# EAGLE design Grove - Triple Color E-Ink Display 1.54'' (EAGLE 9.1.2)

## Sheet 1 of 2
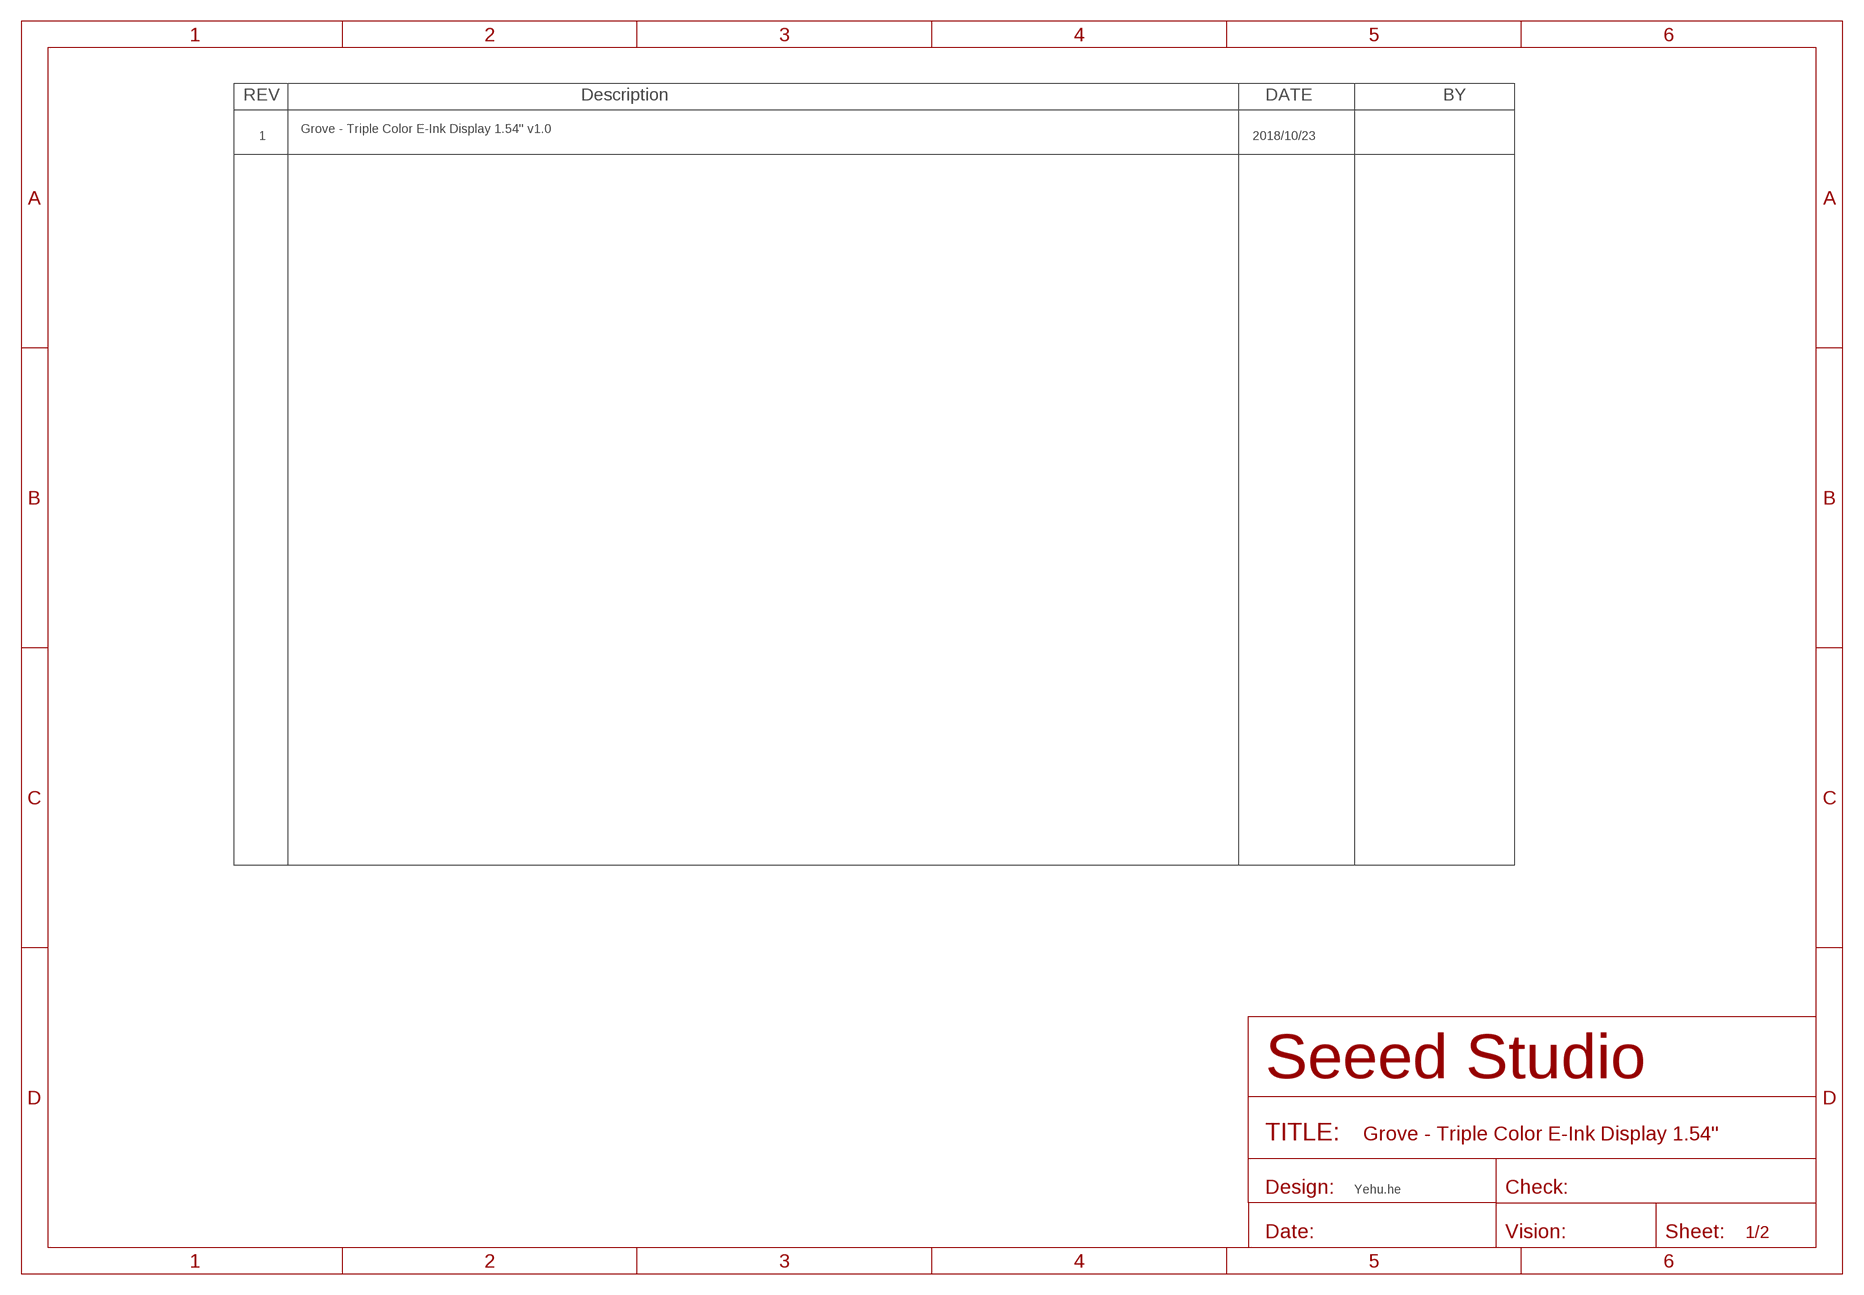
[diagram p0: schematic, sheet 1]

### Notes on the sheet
- Grove - Triple Color E-Ink Display 1.54'' v1.0
- 1 | 2018/10/23
- Yehu.he

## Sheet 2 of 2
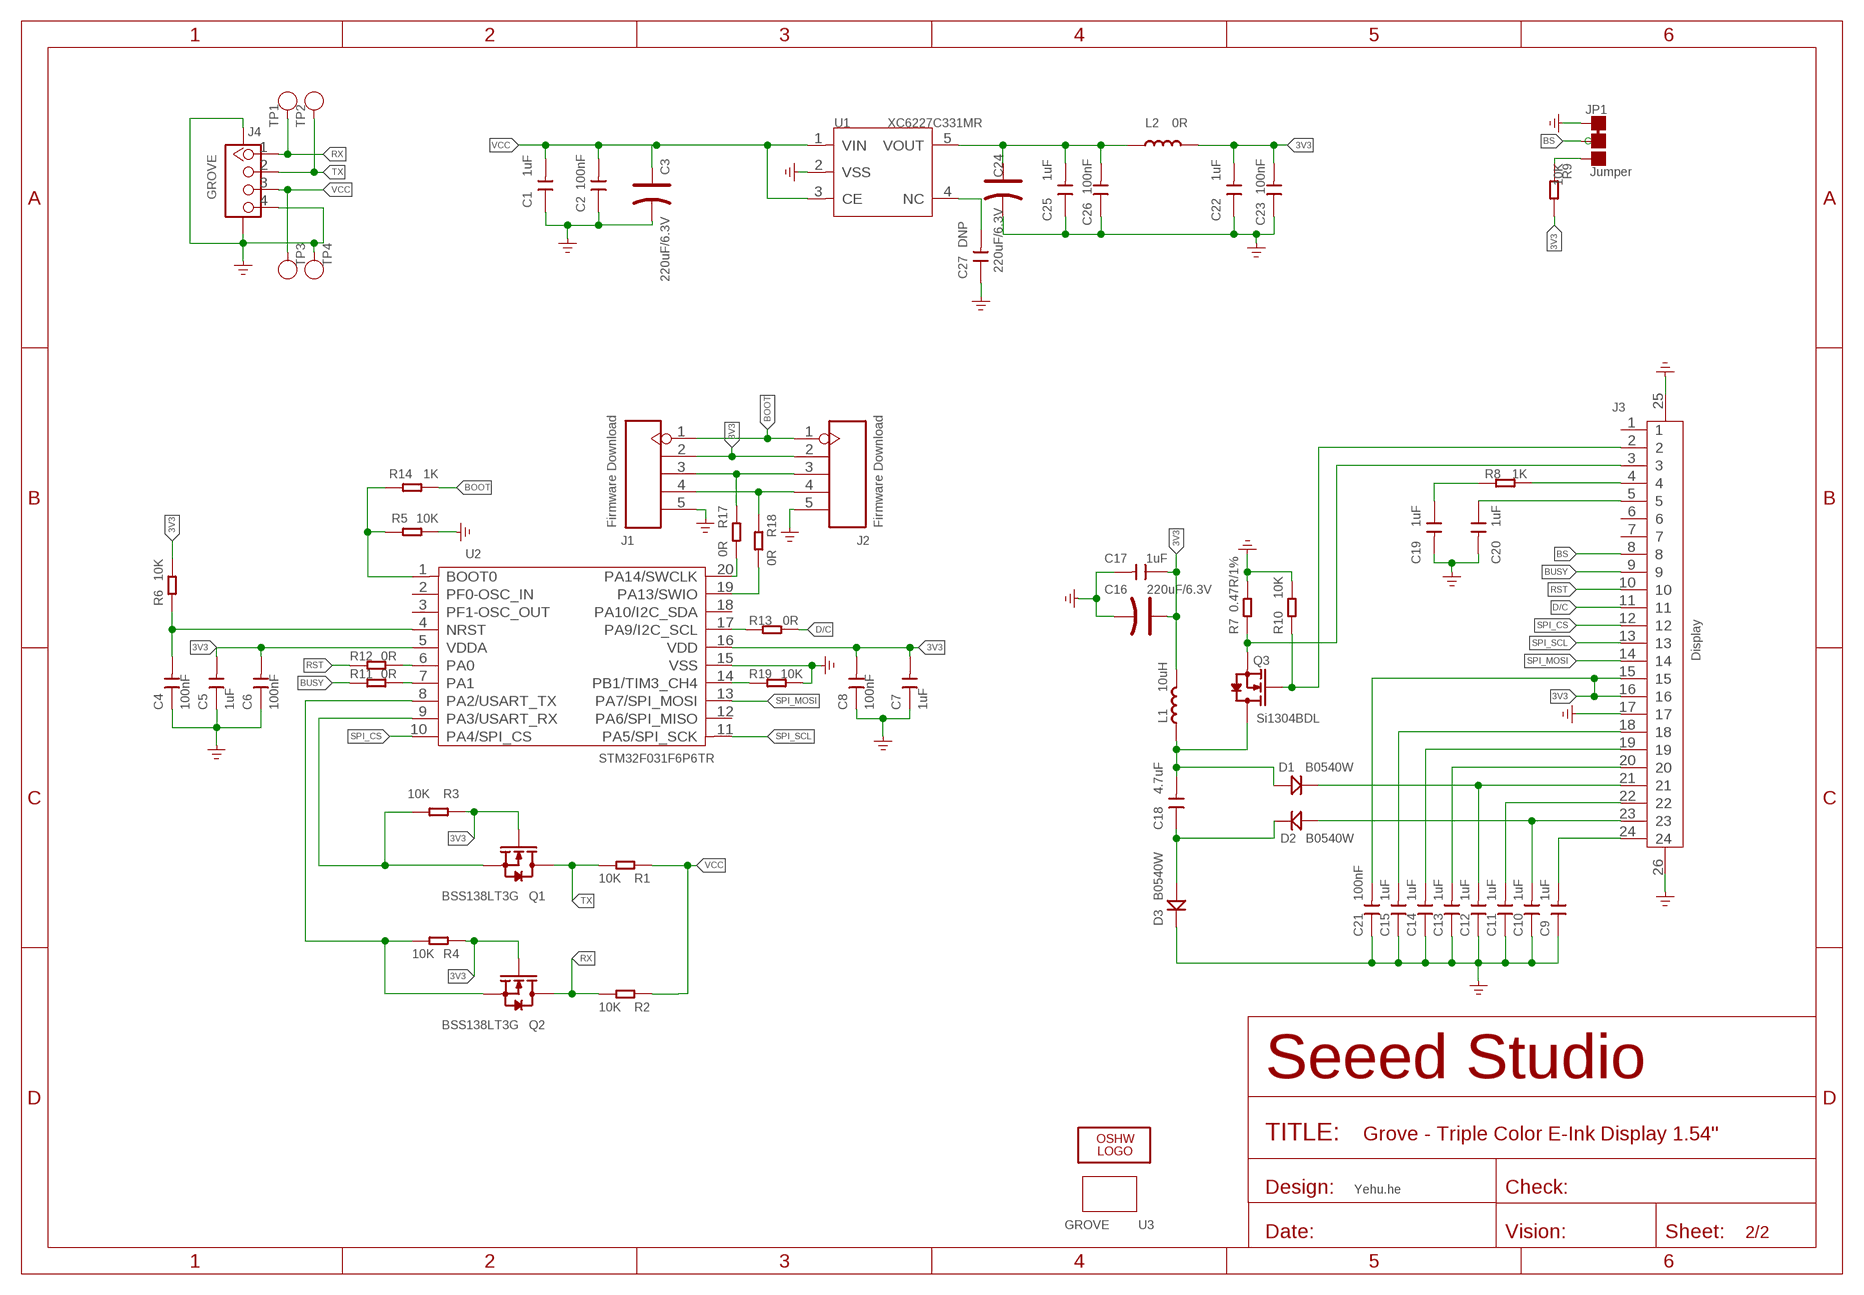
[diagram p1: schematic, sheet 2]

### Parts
C1  1uF  CAP-0603  [C0603]
C2  100nF  CAP-0603  [C0603]
C3  220uF/6.3V  CAP-POLAR-AVX-B  [AVX-B]
C4  100nF  CAP-0603  [C0603]
C5  1uF  CAP-0603  [C0603]
C6  100nF  CAP-0603  [C0603]
C7  1uF  CAP-0603  [C0603]
C8  100nF  CAP-0603  [C0603]
C9  1uF  CAP-0603  [C0603]
C10  1uF  CAP-0603  [C0603]
C11  1uF  CAP-0603  [C0603]
C12  1uF  CAP-0603  [C0603]
C13  1uF  CAP-0603  [C0603]
C14  1uF  CAP-0603  [C0603]
C15  1uF  CAP-0603  [C0603]
C16  220uF/6.3V  CAP-POLAR-AVX-B  [AVX-B]
C17  1uF  CAP-0603  [C0603]
C18  4.7uF  CAP-0805  [C0805]
C19  1uF  CAP-0603  [C0603]
C20  1uF  CAP-0603  [C0603]
C21  100nF  CAP-0603  [C0603]
C22  1uF  CAP-0805  [C0805]
C23  100nF  CAP-0603  [C0603]
C24  220uF/6.3V  CAP-POLAR-AVX-B  [AVX-B]
C25  1uF  CAP-0805  [C0805]
C26  100nF  CAP-0603  [C0603]
C27  DNP  CAP-0603  [C0603]
D1  B0540W  DIODE'0805'  [SOD-323]
D2  B0540W  DIODE'0805'  [SOD-323]
D3  B0540W  DIODE'0805'  [SOD-323]
J1  Firmware Download  HEADER-5P-SMD2.54  [H5-SMD-2.54]
J2  Firmware Download  HEADER-5P-SMD2.54  [H5-SMD-2.54]
J3  Display  FPC-CONNECTOR-24P  [FPCB24-SMD-0.5-17.6X5.0X2MM]
J4  GROVE  GROVE-CONNECTOR-SMD'90D'  [HW4-SMD-2.0-90D]
JP1  Jumper  JP-3P-SHORT  [3P-SMD-SHORT]
L1  10uH  INDUCTOR/FERRITE-BEAD5040S  [L5040S]
L2  0R  INDUCTOR/FERRITE-BEAD'0805'  [L0805]
LOGO2  LOGO-OSHW-FILLX0200-NT  [OSHW_FILLX200_NOTEXT]
Q1  BSS138LT3G  MOSFET-N'SI1304BDL'  [SOT-323]
Q2  BSS138LT3G  MOSFET-N'SI1304BDL'  [SOT-323]
Q3  Si1304BDL  MOSFET-N'SI1304BDL'  [SOT-323]
R1  10K  RES-0603  [R0603]
R2  10K  RES-0603  [R0603]
R3  10K  RES-0603  [R0603]
R4  10K  RES-0603  [R0603]
R5  10K  RES-0603  [R0603]
R6  10K  RES-0603  [R0603]
R7  0.47R/1%  RES-0603  [R0603]
R8  1K  RES-0603  [R0603]
R9  10K  RES-0603  [R0603]
R10  10K  RES-0603  [R0603]
R11  0R  RES-0603  [R0603]
R12  0R  RES-0603  [R0603]
R13  0R  RES-0603  [R0603]
R14  1K  RES-0603  [R0603]
R17  0R  RES-0603  [R0603]
R18  0R  RES-0603  [R0603]
R19  10K  RES-0603  [R0603]
TP1  Test  TEST-POINT'4545'  [TP-D45MIL]
TP2  Test  TEST-POINT'4545'  [TP-D45MIL]
TP3  Test  TEST-POINT'4545'  [TP-D45MIL]
TP4  Test  TEST-POINT'4545'  [TP-D45MIL]
U1  XC6227C331MR  PMIC-LDO-XC6210  [SOT-23-5]
U2  STM32F031F6P6TR  MCU-STM32F030  [TSSOP20-0.65-6.5X4.4MM]
U3  GROVE  GROVE'2X2U'  [GROVE-2*2-DRILL-DIM]

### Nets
3V3: C5.2 C6.2 C7.2 C8.2 C16.+ C17.1 C21.2 C22.2 C23.2 J1.2 J2.2 J3.15 J3.16 L1.2 L2.2 Q1.1(G) Q2.1(G) R3.2 R4.2 R6.1 R9.2 U2.5(VDDA) U2.16(VDD)
123: C24.+ C25.2 C26.2 L2.1 U1.5(VOUT)
BOOT: J1.1 J2.1 R14.1
BS: J3.8 JP1.MM(C)
BUSY: J3.9 R11.1
D/C: J3.11 R13.1
GDR: J3.2 Q3.1(G) R10.1
GND: C1.1 C2.1 C3.- C4.1 C5.1 C6.1 C7.1 C8.1 C9.1 C10.1 C11.1 C12.1 C13.1 C14.1 C15.1 C16.- C17.2 C19.2 C20.2 C21.1 C22.1 C23.1 C24.- C25.1 C26.1 C27.1 D3.- J1.5 J2.5 J3.17 J3.25(P1) J3.26(P2) J4.4 J4.SS1 J4.SS2 JP1.11(L) R5.1 R7.2 R10.2 R19.1 TP4.T U1.2(VSS) U2.15(VSS) ; supply symbol labelled GND_POWER
N$1: R11.2 U2.7(PA1)
N$2: R12.2 U2.6(PA0)
N$3: R13.2 U2.17(PA9/I2C_SCL)
N$4: J1.3 J2.3 R17.1
N$5: R5.2 R14.2 U2.1(BOOT0)
N$6: R19.2 U2.14(PB1/TIM3_CH4)
N$7: C27.2 U1.4(NC)
N$8: C4.2 R6.2 U2.4(NRST)
N$9: C18.1 D2.- D3.+
N$10: J1.4 J2.4 R18.1
N$11: C18.2 D1.+ L1.1 Q3.3(D)
N$12: C19.1 R8.2
N$13: R17.2 U2.20(PA14/SWCLK)
N$14: R18.2 U2.19(PA13/SWIO)
N$22: C15.2 J3.18
N$23: C14.2 J3.19
N$24: C13.2 J3.20
N$25: C12.2 D1.- J3.21
N$26: C11.2 J3.22
N$27: C10.2 D2.+ J3.23
N$28: JP1.00(R) R9.1
RESE: J3.3 Q3.2(S) R7.1
RST: J3.10 R12.1
RX: J4.1 Q2.3(D) R2.1 TP1.T
SCL_3V3: Q1.2(S) R3.1 U2.9(PA3/USART_RX)
SDA_3V3: Q2.2(S) R4.1 U2.8(PA2/USART_TX)
SPI_CS: J3.12 U2.10(PA4/SPI_CS)
SPI_MOSI: J3.14 U2.13(PA7/SPI_MOSI)
SPI_SCL: J3.13 U2.11(PA5/SPI_SCK)
TX: J4.2 Q1.3(D) R1.1 TP2.T
VCC: C1.2 C2.2 C3.+ J4.3 R1.2 R2.2 TP3.T U1.1(VIN) U1.3(CE)
VCOM: C9.2 J3.24
VGH: C20.1 J3.5
VGL: J3.4 R8.1
Unconnected: J3.1 J3.6 J3.7 U2.2(PF0-OSC_IN) U2.3(PF1-OSC_OUT) U2.12(PA6/SPI_MISO) U2.18(PA10/I2C_SDA)

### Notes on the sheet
- Yehu.he

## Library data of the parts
C1 C2 C4-C15 C17-C23 C25-C27 = Discrete-new:CAP: Ceramic Capacitors
C3 C16 C24 = Discrete-new:CAP-POLAR: Electrolytic Capacitors,Tantalum Capacitors and Super Capacitors
D1-D3 = Discrete-new:DIODE*
J1 J2 = Connector-new:HEADER-5P
J3 = Connector-new:FPC-CONNECTOR-24P
J4 = Connector-new:GROVE-CONNECTOR-SMD: 4P-SMD-2.0:320110030;4P-SMD-2.0-90D:320110032
JP1 = Discrete-new:JP-3P-SHORT
L1 L2 = Discrete-new:INDUCTOR/FERRITE-BEAD
LOGO2 = logo:LOGO-OSHW-FILL; PARTNO: DNP
Q1-Q3 = Discrete-new:MOSFET-N: IRLL014: http://www.vishay.com/docs/91319/sihll014.pdf
R1-R14 R17-R19 = Discrete-new:RES
TP1-TP4 = Discrete-new:TEST-POINT; PARTNO: DNP
U1 = IC-new:PMIC-LDO-XC6210
U2 = IC-new:MCU-STM32F030
U3 = moudle-new:GROVE

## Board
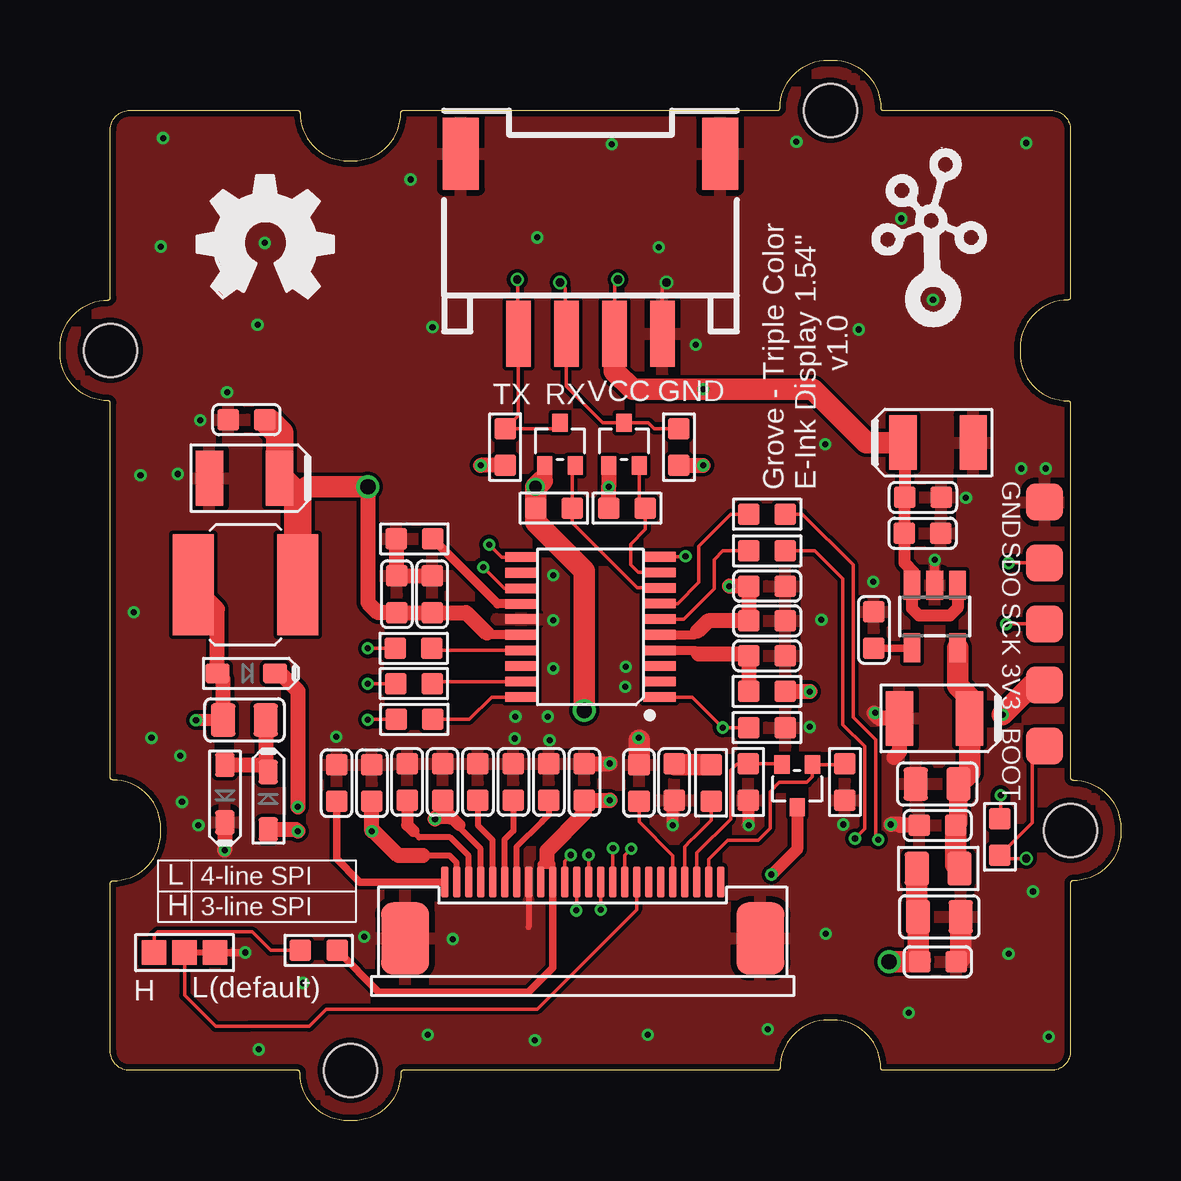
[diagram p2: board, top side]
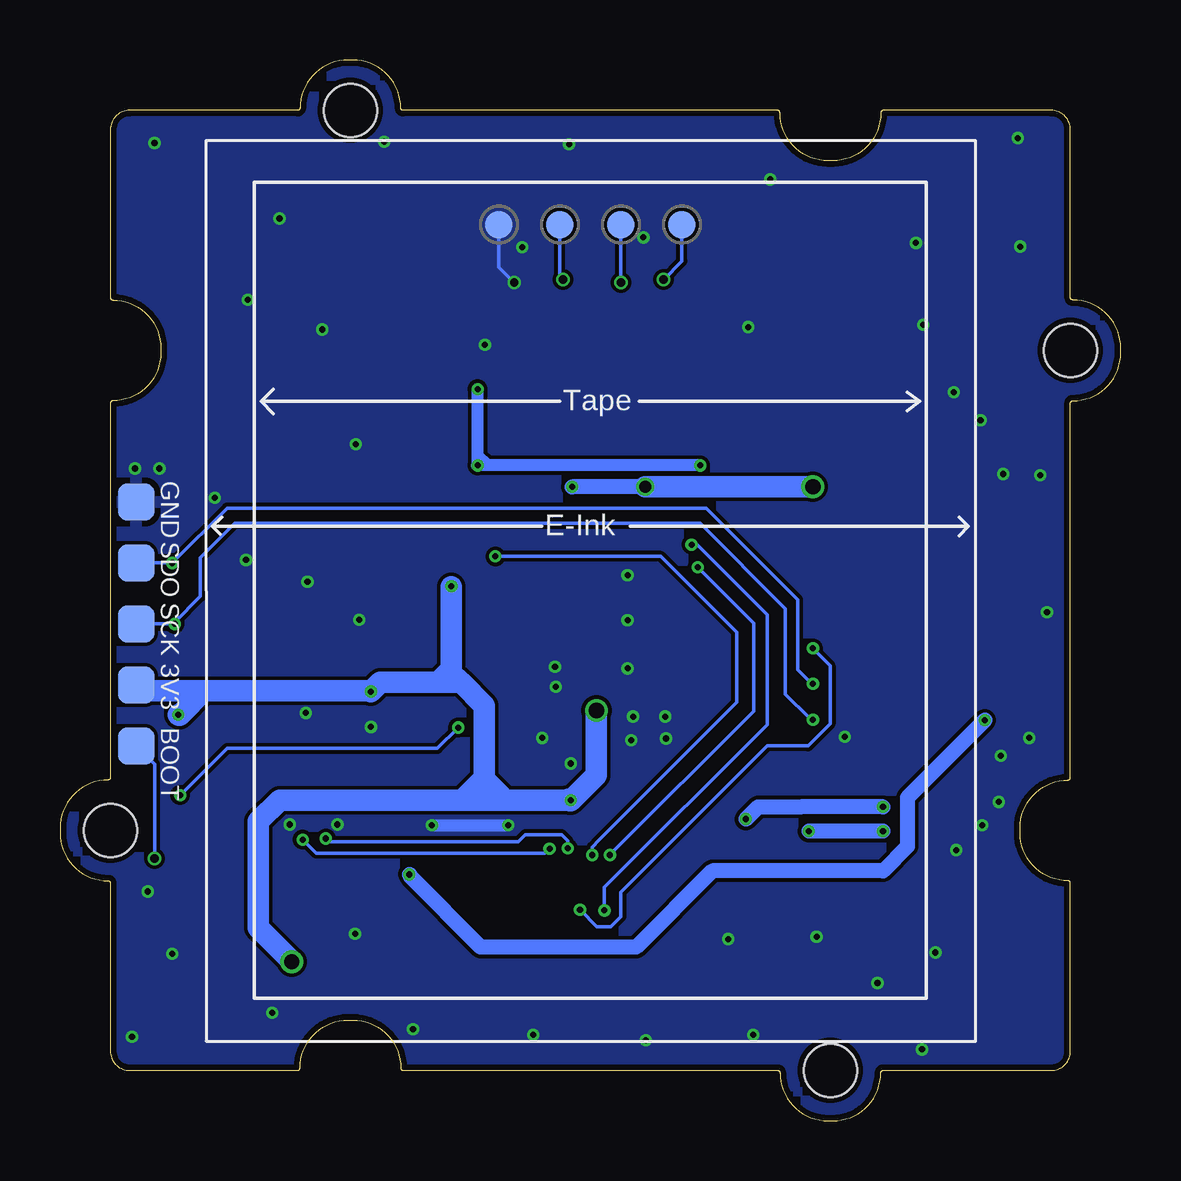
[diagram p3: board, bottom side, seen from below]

Size 44.2 x 44.2 mm. Coordinates in mm from the lower left corner, seen from the top.
Copper layers (1*16): Top 0.035mm / dielectric 1.5mm / Bottom 0.035mm
Design rules "SeeedStudio_2layer_DRU_no_angle_20140221": minimum track width 1mil, minimum drill 10mil, track to track 6mil, track to pad 6mil, pad to pad 6mil, via to via 6mil, smd to smd 0mil, copper to edge 10mil, drill to drill 10mil, minimum pad ring 4mil, minimum via ring 4mil, stop-mask expansion 2mil, vias tented up to drill 25mil, thermal gap 10mil

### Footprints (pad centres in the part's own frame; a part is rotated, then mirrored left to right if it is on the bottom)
C0603 = smd 0.889 x 0.889: 1 -0.762,0; 2 0.762,0
AVX-B = smd 1.143 x 2.286: + 1.46,0; - -1.46,0
C0805 = smd 1.016 x 1.397: 1 -0.889,0; 2 0.889,0
SOD-323 = smd 1 x 0.8: + 1.2,0; - -1.2,0
H5-SMD-2.54 = smd 1.524 x 1.524: 1 0,5.08; 2 0,2.54; 3 0,0; 4 0,-2.54; 5 0,-5.08
FPCB24-SMD-0.5-17.6X5.0X2MM = smd 0.3 x 1.3: 1 5.75,0; 2 5.25,0; 3 4.75,0; 4 4.25,0; 5 3.75,0; 6 3.25,0; 7 2.75,0; 8 2.25,0; 9 1.75,0; 10 1.25,0; 11 0.75,0; 12 0.25,0; 13 -0.25,0; 14 -0.75,0; 15 -1.25,0; 16 -1.75,0; 17 -2.25,0; 18 -2.75,0; 19 -3.25,0; 20 -3.75,0; 21 -4.25,0; 22 -4.75,0; 23 -5.25,0; 24 -5.75,0 | smd 2 x 3: 25 -7.4,-2.35; 26 7.4,-2.35
HW4-SMD-2.0-90D = smd 1.01 x 2.74: 1 -3,-0.1; 2 -1,-0.1; 3 1,-0.1; 4 3,-0.1 | smd 1.5 x 3: SS1 -5.4,7.4; SS2 5.4,7.4
3P-SMD-SHORT = smd 1.016 x 1.016: 00 -1.27,0; 11 1.27,0; MM 0,0
L5040S = smd 1.7 x 4.2: 1 -2.175,0; 2 2.175,0
L0805 = smd 1.016 x 1.397: 1 -0.889,0; 2 0.889,0
SOT-323 = smd 0.762 x 0.635: 1 0.889,-0.635; 2 0.889,0.635; 3 -0.889,0
R0603 = smd 0.889 x 0.889: 1 -0.762,0; 2 0.762,0
TP-D45MIL = smd 1.143 x 1.143: T 0,0
SOT-23-5 = smd 0.69 x 1.2: 1 -0.95,-1.3; 2 0,-1.3; 3 0.95,-1.3; 4 0.95,1.3; 5 -0.95,1.3
TSSOP20-0.65-6.5X4.4MM = smd 0.4 x 1.35: 1 -2.925,-2.875; 2 -2.275,-2.875; 3 -1.625,-2.875; 4 -0.975,-2.875; 5 -0.325,-2.875; 6 0.325,-2.875; 7 0.975,-2.875; 8 1.625,-2.875; 9 2.275,-2.875; 10 2.925,-2.875; 11 2.91,2.875; 12 2.26,2.875; 13 1.61,2.875; 14 0.96,2.875; 15 0.325,2.875; 16 -0.325,2.875; 17 -0.975,2.875; 18 -1.625,2.875; 19 -2.275,2.875; 20 -2.925,2.875
GROVE-2*2-DRILL-DIM = hole 2.2: 10,20; -20,10; -10,-20; 20,-10

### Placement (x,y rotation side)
C1  35.94,24.48 180 top
C2  35.96,25.97 180 top
C3  36.59,28.26 180 top
C4  29.46,19.37 180 top
C5  29.47,20.83 180 top
C6  29.47,22.28 180 top
C7  14.03,21.94 270 top
C8  15.51,21.94 270 top
C9  11.52,14.07 270 top
C10  13,14.07 270 top
C11  14.47,14.12 270 top
C12  15.94,14.12 270 top
C13  17.42,14.12 270 top
C14  18.89,14.12 270 top
C15  20.37,14.12 270 top
C16  7.69,26.78 0 top
C17  7.77,29.22 180 top
C18  7.69,16.7 180 top
C19  25.59,14.12 270 top
C20  24.12,14.08 90 top
C21  21.85,14.12 270 top
C22  36.64,8.5 180 top
C23  36.58,6.62 180 top
C24  36.44,16.77 0 top
C25  36.55,14.03 0 top
C26  36.56,12.31 0 top
C27  33.91,20.45 270 top
D1  7.76,18.64 180 top
D2  8.68,13.34 270 top
D3  6.87,13.63 90 top
J1  41.02,20.7 180 bottom
J2  41.02,20.7 180 top
J3  21.78,9.95 0 top
J4  22.1,32.9 0 top
JP1  5.19,7 0 top
L1  7.73,22.33 0 top
L2  36.59,10.51 180 top
LOGO2  5.72,34.29 0 top
Q1  23.5,28.2 270 top
Q2  20.83,28.2 270 top
Q3  30.71,13.96 90 top
R1  25.78,28.07 270 top
R2  18.54,28.07 270 top
R3  23.62,25.53 180 top
R4  20.58,25.53 180 top
R5  29.46,16.39 180 top
R6  29.46,17.89 180 top
R7  28.68,14.12 270 top
R8  27.13,14.08 90 top
R9  10.78,7.1 0 top
R10  32.7,14.12 270 top
R11  29.47,25.28 180 top
R12  29.47,23.75 180 top
R13  14.73,19.69 0 top
R14  39.16,11.83 90 top
R17  14.76,16.72 0 top
R18  14.75,18.21 0 top
R19  14.77,24.25 0 top
TP1  18.29,37.34 90 bottom
TP2  20.83,37.34 90 bottom
TP3  23.37,37.34 90 bottom
TP4  25.91,37.34 90 bottom
U1  36.45,21.01 180 top
U2  22.1,20.58 90 top
U3  22.1,22.1 0 top
U$20  [GROVE-SILK-BIG]  36.32,34.04 0 top

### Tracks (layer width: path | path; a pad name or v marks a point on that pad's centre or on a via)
3V3  (via drill 0.25 pad 0.51, 0.51 pad 0.51, 0.64 pad 0.51)
  Top 0.152: C17.1 8.52,29.22 8.51,29.21
  Top 0.254: J3.15 20.53,10.72 20.45,10.8 20.3,10.8 20.12,10.8 20.03,10.71 J3.16
  Top 0.305: J3.15 20.53,6.38 19.51,5.36 14.1,5.36 13.28,5.36 R9.2
  Top 0.381: U2.16 17.85,20.25 17.78,20.32 17.4,20.7 | U2.5 26.42,20.25 26.57,20.4
  Top 0.508: 35.84,6.68 35.84,6.65 C23.2 | C22.2 35.77,8.49
  Top 0.635: 17.78,20.32 16.93,21.18 C8.2 C7.2 13.24,21.18 12.83,21.59 v12.83,26.42 | R3.2 v22.86,26.42 Q1.1 | R4.2 v19.81,26.42 20.2,26.8 Q2.1 | 26.57,20.4 27,20.83 C5.2 C6.2 v27.89,22.28 | 20.3,10.8 20.3,11.26 21.85,12.82 C21.2 v22.91,13.36 | R6.1 31.23,17.89 v31.24,17.88 | 8.71,29.09 8.64,29.09 8.51,29.21 | 10.31,26.42 9.91,26.02
  Top 0.889: v12.83,26.42 10.31,26.42 | v21.85,17.1 21.85,22.91 19.81,24.95 R4.2 19.81,26.39 20.09,26.67 | L2.2 35.7,8.55 35.77,8.49 | C22.2 35.75,6.77 35.84,6.68 35.82,6.68 35.77,6.63 v34.55,6.63 | J1.2 40.52,18.16 v39.27,16.92
  Top 1.143: L1.2 9.91,26.02 C16.+ 9.15,28.65 8.71,29.09
  Bottom 0.152: 22.91,13.34 v22.91,13.36
  Bottom 0.254: 27.89,19.08 28.09,19.08 28.86,18.32
  Bottom 0.635: v19.81,26.42 v22.86,26.42 | v27.89,22.28 27.89,22.25 | 27.89,21.31 27.89,21.24
  Bottom 0.889: v19.81,26.42 v12.83,26.42 | v21.85,17.1 21.85,14.4 22.91,13.34 22.96,13.34 23.01,13.39 | v22.91,13.36 26.6,13.36 | 26.6,13.36 35.05,13.36 35.94,12.47 35.94,8.05 34.6,6.71 34.6,6.68 v34.55,6.63 | 27.48,18.27 27.89,18.67 27.89,19.08 27.89,21.31 27.89,22.25 | 27.48,18.27 26.52,17.3 26.52,14.23 | 26.52,14.23 26.52,14.2 | 26.52,14.2 26.52,13.44 26.6,13.36 | 27.48,18.27 30.86,18.27 31.22,17.91 | 31.22,17.91 v31.24,17.88 | 31.22,17.91 38.2,17.91 | 38.2,17.91 39.22,16.89 39.25,16.89 v39.27,16.92 | 26.52,14.2 26.49,14.2 25.83,13.54 | 26.52,14.23 26.57,14.23 27.33,13.46 | 38.2,17.91 40.77,17.91 J1.2
123
  Top 0.762: C25.2 37.44,12.42 C26.2
  Top 0.889: U1.5 37.4,18.13 37.9,17.63 37.9,16.79 37.92,16.77 C24.+ 37.9,14.58 | 37.9,14.58 37.87,14.56 | 37.9,14.58 37.9,14.5 37.42,14.02 37.43,14.02 C25.2 | C26.2 37.33,10.67 L2.1
BOOT  (via drill 0.35)
  Top 0.152: J1.1 40.52,15.12 40.52,12.42 R14.1 39.3,10.92 v40.26,10.92
  Bottom 0.152: v40.26,10.92 40.26,14.86 J1.1
BS
  Top 0.152: J3.8 24.03,8.8 19.88,4.65 11.1,4.65 10.38,3.93 7.88,3.93 | 7.88,3.93 7.83,3.93 | JP1.MM 5.19,5.23 6.49,3.93 7.88,3.93
BUSY  (via drill 0.25 pad 0.51)
  Top 0.152: R11.1 30.93,25.28 33.05,23.16 33.05,16.82 33.99,15.88 33.99,11.81 v34.09,11.71 | J3.9 23.53,11.06 v23.8,11.33
  Bottom 0.152: v23.8,11.33 23.83,11.33 24.01,11.15 33.53,11.15 v34.09,11.71
D/C  (via drill 0.25 pad 0.51)
  Top 0.152: R13.1 v12.83,19.69 | J3.11 v22.53,8.79
  Bottom 0.152: v12.83,19.69 12.11,18.97 12.11,16.54 13.03,15.62 14.73,15.62 20.83,9.53 20.83,8.51 21.25,8.09 21.83,8.09 v22.53,8.79
GDR
  Top 0.152: J3.2 27.03,10.9 27.82,11.69 29.09,11.69 29.59,12.19 29.59,13.72 29.97,14.1 31.12,14.1 31.35,14.33 Q3.1 32.67,14.84 R10.1
GND  (via drill 0.25 pad 0.51, 0.35)
  Top 0.152: JP1.11 6.78,7.01 | v7.72,7.01 | J4.4 25.1,34.75 v25.28,34.93
  Top 0.254: J3.17 19.53,8.08
  Top 0.305: JP1.11 v7.72,7.01
  Top 0.381: U1.2 v36.45,23.37
  Top 0.508: R7.2 28.68,12.35 v28.7,12.32 | v25.53,12.32 25.53,13.3 C19.2
  Top 0.635: R19.1 14,22.73 C7.1 C8.1 | C21.1 v22.91,14.88 v22.91,14.89 | D3.- 6.87,11.44 v6.86,11.28 | 34.75,15.14 34.98,15.37 C24.- 34.14,16.77 33.91,17 | C26.1 35.02,12.31 34.95,12.37 34.95,12.35 v34.62,12.35
  Top 0.889: C22.1 37.53,6.81 C23.1 | C20.2 24.12,15.85 24.13,15.85
  Bottom 0.152: v25.28,34.93 25.91,35.56 TP4.T
  Bottom 0.508: v28.7,12.32 v25.53,12.32
  other vias: 16.36,7.57 12.68,7.67 5.08,13.29 5.01,15.22 15.32,3.58 24.49,3.58 19.79,3.35 29.49,3.81 31.9,7.8 35.36,4.5 41.2,3.51 39.52,6.96 40.54,9.55 33.89,22.46 37.75,25.96 31.88,28.2 24.94,36.4 36.37,34.22 30.69,40.79 40.26,40.74 35.05,37.59 22.99,40.69 14.61,39.22 15.52,33.07 8.23,33.17 4.29,40.95 8.54,36.58 4.19,36.43 5.84,29.19 3.35,26.9 3.08,21.19 3.81,15.95 4.9,26.95 6.96,30.36 23.57,18.93 20.55,20.86 20.55,22.74 20.55,18.85 23.55,18.09 31.24,16.41 20.4,15.85 18.95,15.93 11.51,16 5.77,12.32 24.11,15.95 32.64,12.35 33.96,16.99 31.73,20.88 18.98,16.84 20.32,16.84 19.89,36.81 26.49,32.34 33.28,32.97 41.07,27.18 40.06,27.18 10.14,5.74 8.28,2.97
  pour Top: 0.13,46.84 43,46.84 46.18,43.66 46.18,1.98 43.64,-0.56 0.18,-0.56 -2.49,2.11 -2.49,44.2 0.13,46.81
  pour Bottom: 1.75,46.1 42.09,46.1 45.11,43.08 45.11,2.8 42.55,0.23 1.55,0.23 -1.27,3.05 -1.27,43.08
N$1
  Top 0.152: U2.7 25.74,21.55 26.62,22.43 26.62,23.94 27.96,25.28 R11.2
N$2
  Top 0.152: R12.2 27.62,23.75 27.26,23.39 27.26,22.18 26.36,21.27 26.32,21.24 25.98,20.9 U2.6
N$3
  Top 0.152: U2.17 15.58,19.6 R13.2
N$4  (via drill 0.25 pad 0.51)
  Top 0.152: R17.1 v12.84,16.72 v12.83,16.72 | v39.42,20.7 40.9,20.7 40.97,20.63 40.97,20.65 J1.3
  Bottom 0.152: v12.83,16.72 12.83,16.77 12.96,16.77 13.97,17.78 13.97,21.34 17.53,24.89 27.56,24.89 36.91,24.89 38.36,23.45 38.36,21.85 39.42,20.78 v39.42,20.7 J1.3
N$5  (via drill 0.25 pad 0.51)
  Top 0.152: R5.2 v27.61,16.39 26.35,17.65 U2.1 | 39.2,13.56 v39.19,13.57 39.19,12.62 R14.2
  Bottom 0.152: 39.19,13.54 v39.19,13.57 37.24,15.52 28.48,15.52 v27.61,16.39
N$6
  Top 0.381: U2.14 18.24,21.54 R19.2
N$7
  Top 0.305: C27.2 35.47,19.69 U1.4
N$8
  Top 0.152: C4.2 28.7,19.35 28.68,19.33
  Top 0.381: U2.4 26.45,19.6 26.6,19.46
  Top 0.635: 26.6,19.46 28.55,19.46 28.68,19.33 | C4.2 R6.2
N$9
  Top 0.635: D3.+ 8.38,14.83 D2.- 8.68,14.52 8.64,14.48 8.58,14.54 C18.1
N$10  (via drill 0.25 pad 0.51)
  Top 0.152: R18.1 v12.83,18.21 | v39.52,23.24 40.92,23.24 40.95,23.27 40.95,23.22 41.02,23.22 | 41.02,23.22 40.97,23.27 | 41.02,23.22 J1.4
  Bottom 0.152: v12.83,18.21 12.88,18.21 13.46,18.8 13.46,21.72 17.27,25.53 27.31,25.53 37.24,25.53 39.5,23.27 v39.52,23.24 J1.4
N$11  (via drill 0.25 pad 0.51)
  Top 0.152: Q3.3 30.71,11.33 v29.64,10.26 | v5.67,16.69 6.79,16.69 C18.2
  Top 0.508: C18.2 v5.68,16.7 v5.67,16.69 | Q3.3 30.71,11.31 29.67,10.26
  Top 0.635: C18.2 6.8,18.41 D1.+ 6.56,21.33 L1.1
  Bottom 0.635: v5.67,16.69 8.89,13.46 8.89,11.43 9.91,10.42 17.02,10.42 20.2,7.24 26.67,7.24 29.59,10.16 29.59,10.21 v29.64,10.26
N$12
  Top 0.152: 25.61,14.86 25.6,14.86 C19.1
  Top 0.889: R8.2 25.62,14.84 25.61,14.86
N$13
  Top 0.152: U2.20 17.98,17.65 17.05,16.72 R17.2
N$14
  Top 0.152: U2.19 15.6,18.3 R18.2
N$22
  Top 0.254: J3.18 19.03,11.41 20.07,12.45 20.14,12.52 20.37,12.75 C15.2
N$23
  Top 0.254: J3.19 18.53,11.72 18.89,12.08 C14.2
N$24
  Top 0.254: C13.2 17.42,12.31 17.91,11.81 17.93,11.79 18.03,11.69 J3.20
N$25  (via drill 0.25 pad 0.51)
  Top 0.254: J3.21 17.53,11.33 16.26,12.6 15.94,12.92 C12.2
  Top 0.508: C12.2 15.94,13.02 16.64,12.32 | 16.26,12.6 15.65,12.6 v15.62,12.58
  Top 0.635: D1.- 9.17,18.64 9.91,17.91 v9.91,13.08 | C12.2 15.94,12.89 v15.62,12.58
  Bottom 0.152: 13.46,13.08 13.34,13.08
  Bottom 0.635: v9.91,13.08 13.34,13.08 | v15.62,12.58 15.12,13.08 13.46,13.08
N$26
  Top 0.254: C11.2 14.47,12.31 14.96,11.81 16.26,11.81 17.03,11.04 J3.22
  Top 0.508: C11.2 14.47,12.34 14.73,12.07
N$27  (via drill 0.25 pad 0.51)
  Top 0.254: J3.23 16.53,10.75 16.23,11.05 15.12,11.05
  Top 0.635: 13.01,13.3 C10.2 v13,12.07 13.08,12.07 14.1,11.05 15.12,11.05 | D2.+ 9.84,12.14 v9.91,12.07
  Bottom 0.635: v9.91,12.07 v13,12.07
N$28
  Top 0.152: R9.1 8.78,7.1 8,7.88 4.07,7.88 3.92,7.73 JP1.00
RESE
  Top 0.152: J3.3 26.53,11.16 27.94,12.58 27.94,14.61 28.2,14.86 28.66,14.86 R7.1 30.05,14.88 Q3.2
RST  (via drill 0.25 pad 0.51)
  Top 0.152: R12.1 31.45,23.75 32.62,22.59 32.62,16.51 33.53,15.6 33.53,12.17 v33.12,11.76 | J3.10 23.03,11.35 v23.04,11.36
  Bottom 0.152: v23.04,11.36 23.04,11.66 23.3,11.92 24.81,11.92 25.1,11.64 33,11.64 v33.12,11.76
RX  (via drill 0.35)
  Top 0.152: Q2.3 20.58,28.83 R2.1 19.1,29.39 J4.1 19.08,32.8 19.08,32.79 19.08,35.03 v19.05,35.05
  Top 0.508: 19.08,32.79 19.05,32.77
  Bottom 0.152: v19.05,35.05 18.29,35.82 TP1.T
SCL_3V3
  Top 0.152: Q1.2 24.13,25.78 R3.1 24.39,24.64 23.77,24.03 23.77,23.17 24.09,22.85 U2.9
SDA_3V3
  Top 0.152: U2.8 24.05,22.2 21.34,24.92 R4.1 21.34,27.18 Q2.2
SPI_CS  (via drill 0.25 pad 0.51)
  Top 0.152: U2.10 26.04,23.5 v26.06,23.52 | J3.12 v22.03,11.07 v22.02,11.08
  Bottom 0.152: v26.06,23.52 19.16,23.52 16,20.36 16,17.43 21.74,11.69 22.02,11.41 v22.02,11.08
SPI_MOSI  (via drill 0.25 pad 0.51)
  Top 0.152: U2.13 18.51,22.19 v17.63,23.07 | J3.14 21.03,10.82 v21.29,11.08
  Bottom 0.152: v17.63,23.07 15.29,20.73 15.29,17.07 v21.29,11.08
SPI_SCL  (via drill 0.25 pad 0.51)
  Top 0.152: U2.11 18.4,23.49 v17.88,24.01 | J3.13 21.53,8.78 v21.52,8.77
  Bottom 0.152: v21.52,8.77 21.52,9.73 14.73,16.51 14.73,21.08 17.66,24.01 v17.88,24.01
TX  (via drill 0.35)
  Top 0.152: R1.1 24.77,28.83 24.51,29.09 Q1.3 22.61,29.09 21.08,30.61 21.08,32.78 J4.2 21.11,32.87 | 21.06,32.92 21.06,34.7 v20.83,34.93
  Top 0.508: 21.11,32.87 21.06,32.92
  Bottom 0.152: v20.83,34.93 TP2.T
VCC  (via drill 0.25 pad 0.51, 0.35)
  Top 0.152: J4.3 23.12,32.81 23.12,32.92 23.12,34.93 v23.24,35.05
  Top 0.508: 23.12,32.92 23.14,32.9 | U1.1 37.4,21.37 37.09,21.06 35.79,21.06 35.5,21.35 U1.3 35.56,22.38 35.56,22.86 35.18,23.24 C1.2 35.18,25.96 C2.2 35.2,28.2 C3.+
  Top 0.635: R2.2 v17.53,27.31 | R1.2 v26.8,27.31
  Top 0.889: J4.3 23.1,31.24 23.85,30.48 v26.8,30.48 31.37,30.48 33.59,28.26 C3.+
  Bottom 0.152: v23.24,35.05 23.37,35.18 TP3.T
  Bottom 0.254: 26.8,27.87 26.77,27.87 26.24,27.33
  Bottom 0.508: v17.53,27.31 v26.8,27.31 | v26.8,27.31 26.82,27.31 | v26.8,27.31 26.8,27.87 v26.8,30.48
VCOM
  Top 0.305: C9.2 11.52,10.91 12.42,10.01 12.45,9.98 12.48,9.95 J3.24
VGH
  Top 0.152: C20.1 24.12,12.46 25.53,11.05 J3.5
VGL
  Top 0.152: R8.1 27.13,12.52 26.42,11.81 26.29,11.69 26.03,11.43 J3.4

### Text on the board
bPlace: Tape | E-Ink
tNames: TX | RX | VCC | GND | GND | Grove - Triple Color / E-Ink Display 1.54'' / v1.0 | SDO | SCK | 3V3 | BOOT | L | 4-line SPI | H | 3-line SPI | H | L(default)
bNames: GND | SDO | SCK | 3V3 | BOOT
